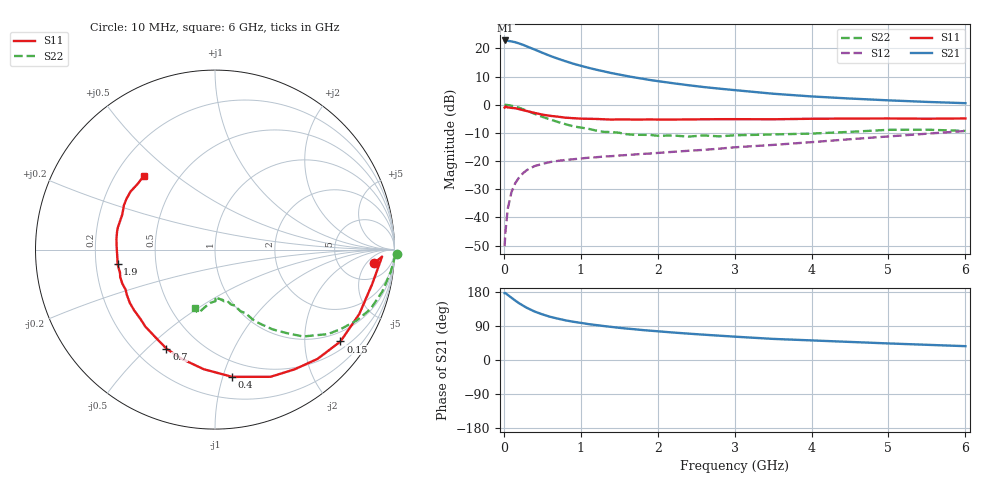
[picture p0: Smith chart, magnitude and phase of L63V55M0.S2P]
!  INFINEON TECHNOLOGIES Small Signal Semiconductors
! BFR380L3 , Si-NPN RF-Transistor in TSLP-3-1
!  Vce=3.5 V,  Ic=5 mA
! Common Emitter S-Parameters:  07. March 2005
#  GHz  S  MA  R  50
! f  S11  S21  S12  S22
! GHz  Mag  Ang  Mag  Ang  Mag  Ang  Mag  Ang
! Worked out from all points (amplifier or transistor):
!   36 points, 10 MHz to 6 GHz, reference 50 ohm
!   highest |S21| = 22.8 dB at 20 MHz (marker M1)
!   |S21| within 3 dB of that: start of sweep to 379.7 MHz
!   unconditionally stable (mu >= 1): 2.526 GHz to 4.656 GHz
!   at 250 MHz: K = 0.17, MSG = 22.8 dB, |S12| = -24.3 dB
!   at 1.4 GHz: K = 0.75, MSG = 14.7 dB, |S12| = -18.2 dB
!   at 6 GHz: K = 0.93, MSG = 4.9 dB, |S12| = -9.3 dB
!   S11 on the Smith chart (normalised r, x): 10 MHz: 11, -8; 150 MHz: 0.71, -2.90; 400 MHz: 0.37, -1.07; 700 MHz: 0.32, -0.58; 1.9 GHz: 0.29, -0.07; 6 GHz: 0.32, +0.39
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0.01  0.89 -4.9  13.76 176.7  0.0031 87.3  1.012 -1.5
0.02  0.9317 -2.4  13.82 176.9  0.0054 92.2  0.9998 -3.1
0.05  0.8968 -12.3  13.63 171.9  0.0141 85.3  0.987 -7.2
0.1  0.8805 -24.0  13.27 164.2  0.0285 78.1  0.9605 -14.2
0.15  0.8664 -36.2  12.84 156.6  0.041 71.4  0.9271 -21.0
0.2  0.8351 -46.8  12.2 149.5  0.0518 66.6  0.8832 -26.5
0.25  0.801 -56.4  11.54 143.5  0.0612 61.4  0.8307 -32.1
0.3  0.7733 -66.4  10.82 137.6  0.0695 58.3  0.786 -36.8
0.4  0.7156 -82.3  9.533 127.9  0.0817 52.0  0.6894 -44.6
0.5  0.6692 -95.4  8.368 120.5  0.0893 48.1  0.6112 -49.5
0.6  0.636 -107.2  7.372 114.1  0.0962 44.9  0.5489 -54.1
0.7  0.6145 -116.1  6.582 109.2  0.101 43.4  0.4961 -57.7
0.9  0.5782 -132.2  5.363 101.0  0.1079 41.6  0.4144 -63.1
1.1  0.5635 -142.9  4.523 94.7  0.1148 41.4  0.3743 -67.2
1.5  0.5501 -159.9  3.432 84.9  0.1256 42.9  0.3186 -73.7
1.9  0.549 -171.6  2.751 77.4  0.1364 45.6  0.2921 -80.1
2.2  0.5463 -178.5  2.409 72.5  0.1461 48.0  0.2849 -81.9
2.8  0.5548 169.7  1.931 64.2  0.1663 52.7  0.2748 -89.4
3.5  0.5523 159.2  1.569 55.7  0.1939 55.7  0.297 -94.7
4.5  0.5685 150.2  1.289 47.7  0.2445 60.1  0.3304 -100.6
5.5  0.5653 140.0  1.123 40.1  0.3065 60.8  0.361 -106.2
6  0.5716 133.8  1.066 36.5  0.3424 59.9  0.3434 -108.9
